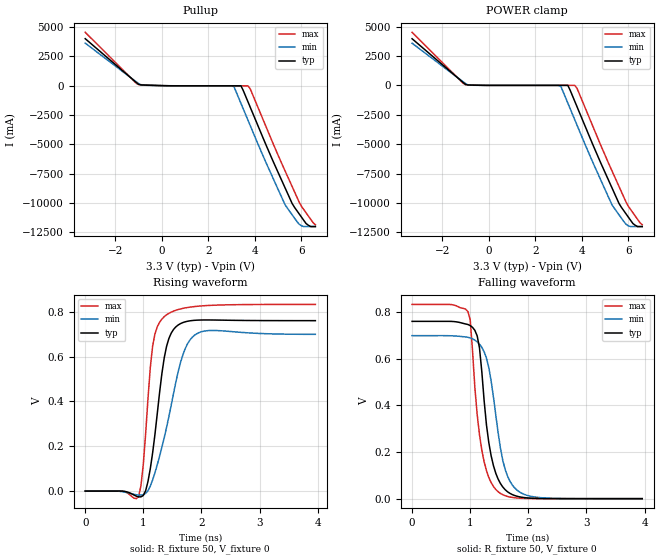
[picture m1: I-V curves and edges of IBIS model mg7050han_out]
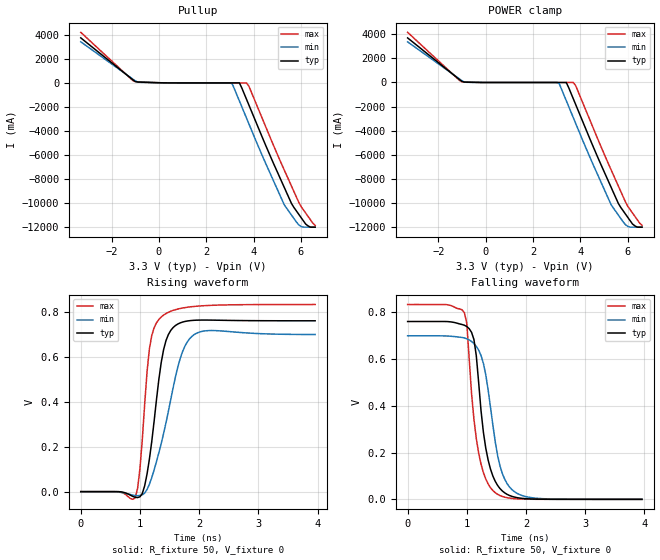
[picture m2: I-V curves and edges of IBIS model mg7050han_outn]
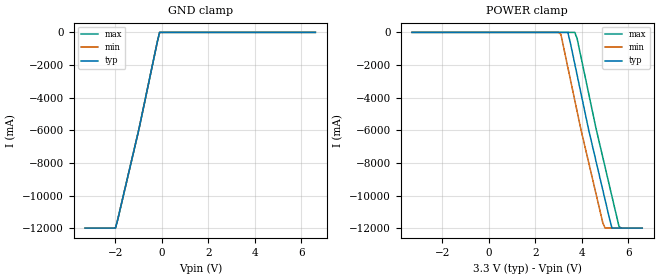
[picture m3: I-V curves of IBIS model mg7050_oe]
|   IBIS File mg7050han_4a_33v_100.ibs  ZSEL=H(ZO=100ohm)
[IBIS Ver]   3.2
[Comment Char]   |_char
[File name]   mg7050han_4a_33v_100.ibs
[File Rev]   1.0
[Date]   Jan 23, 2014
[Source]
|   Component MG7050HAN HCSL 4-OUTPUT 3.3V
[Component]   mg7050han-hcsl-4out-100ohm
[Manufacturer]   Seiko Epson Corporation
[Package]
| variable   typ   min   max
R_pkg   0.27   NA   NA
L_pkg   1.66n   NA   NA
C_pkg   0.53p   NA   NA
[Pin]   signal_name   model_name   R_pin   L_pin   C_pin
1   vcc1   POWER   NA   NA   NA
2   out1p   mg7050han_out   0.34   2.1nH   0.58pF
3   out1n   mg7050han_outn  0.25   1.5nH   0.50pF
4   out2p   mg7050han_out   0.22   1.3nH   0.44pF
5   out2n   mg7050han_outn  0.25   1.7nH   0.59pF
6   zsel   mg7050_zsel   NA   NA   NA
7   oe   mg7050_oe   NA   NA   NA
8   out3n   mg7050han_outn  0.25   1.7nH   0.62pF
9   out3p   mg7050han_out   0.22   1.3nH   0.49pF
10   out4n   mg7050han_outn  0.25   1.5nH   0.46pF
11   out4p   mg7050han_out   0.34   2.1nH   0.57pF
12   vcc2   POWER   NA   NA   NA
13   vcc   POWER   NA   NA   NA
14   gnd   GND   NA   NA   NA
[Diff Pin] inv_pin vdiff   tdelay_typ
2   3   0   0
4   5   0   0
9   8   0   0
11   10   0   0
| Models and submodels in the file (4): mg7050han_out (Open_source), mg7050han_outn (Open_source), mg7050_oe (Input), mg7050_zsel (Input)
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[Model]   mg7050han_out
Model_type Open_source
Enable Active-High
Polarity Non-Inverting
Vref=0
Vmeas=0.375
Rref=50
Cref=0
C_comp   4.79p   4.56p   5.00p
[Temperature Range] 25   85   -40
[Voltage Range]   3.3   2.97   3.63
[POWER Clamp Reference]3.3   2.97   3.63
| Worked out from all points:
|   slope of the pullup table from 0 to 0.495 V, typ, clamps not added: 36.3 ohm
|   POWER clamp passes 1 mA (typ) near -0.12 V on its own axis
|   falling waveform, R_fixture 50, V_fixture 0: 20-80 % time 215ps typ, 264ps min, 203ps max; typ from 0.761 V to 0 V
|   rising waveform, R_fixture 50, V_fixture 0: 20-80 % time 221ps typ, 363ps min, 161ps max; typ from 0 V to 0.761 V
[Pullup]
-3.3V     4.003A     3.625A     4.547A
-1V       105.9mA    168.5mA    94.6mA
3V        -15.26mA   -14.11mA   -16.67mA
3.1V      -15.26mA   -92.55mA   -16.7mA
3.4V      -15.27mA   -1.516A    -16.77mA
3.7V      -1.374A    -2.939A    -16.79mA
3.8V      -1.849A    -3.414A    -283.8mA
5.3V      -8.729A    -10.17A    -7.282A
5.6V      -10.05A    -11.01A    -8.598A
6V        -11.2A     -11.95A    -10.28A
6.3V      -11.91A    -12.01A    -11.12A
6.6V      -12.02A    -12.01A    -11.87A
[POWER Clamp]
-3.3V     3.964A     3.584A     4.512A
-1V       82.86mA    152.1mA    62.75mA
3V        -215.5pA   -247.8pA   -192.8pA
3.1V      -226.7pA   -83.17mA   -204pA
3.4V      -260.3pA   -1.507A    -237.6pA
3.7V      -1.364A    -2.93A     -271.3pA
3.8V      -1.839A    -3.405A    -272.9mA
5.3V      -8.719A    -10.16A    -7.271A
5.6V      -10.03A    -11A       -8.587A
6V        -11.19A    -11.94A    -10.27A
6.3V      -11.89A    -12A       -11.11A
6.6V      -12A       -12A       -11.85A
[Falling Waveform]
R_fixture=50
V_fixture=0
V_fixture_min=0
V_fixture_max=0
0s        760.7mV    699.5mV    833.4mV
960ps     747.2mV    692.4mV    802.9mV
1ns       742.6mV    689.8mV    767.4mV
1.12ns    698.5mV    672.8mV    361.2mV
1.2ns     544.1mV    648.9mV    208.1mV
1.32ns    240.8mV    562.5mV    91.12mV
1.48ns    84.18mV    283.9mV    29.88mV
1.64ns    30.11mV    98.17mV    9.663mV
1.92ns    4.964mV    19.44mV    1.33mV
3.96ns    0V         2.633uV    0V
[Rising Waveform]
R_fixture=50
V_fixture=0
V_fixture_min=0
V_fixture_max=0
0s        851.7nV    1.086uV    0V
920ps     -26.05mV   -17.89mV   -23.44mV
1ns       -19.53mV   -15.94mV   120.9mV
1.12ns    100.1mV    22.23mV    551.4mV
1.16ns    170.5mV    49.57mV    646.9mV
1.36ns    595.2mV    238.7mV    778.6mV
1.48ns    705.2mV    383.7mV    798.9mV
1.64ns    747.6mV    574.2mV    813.2mV
1.88ns    762.3mV    695.6mV    823.7mV
3.96ns    760.7mV    699.6mV    833.3mV
[Ramp]
R_load=50
dV/dt_r   4.564E-1/2.190E-10   4.197E-1/3.615E-10   5.000E-1/1.571E-10
dV/dt_f   4.564E-1/2.120E-10   4.197E-1/2.622E-10   5.000E-1/1.998E-10
|[End   mg7050han_out
[Model]   mg7050han_outn
Model_type Open_source
Enable Active-High
Polarity Inverting
Vref=0
Vmeas=0.375
Rref=50
Cref=0
C_comp   4.79p   4.56p   5.00p
[Temperature Range] 25   85   -40
[Voltage Range]   3.3   2.97   3.63
[POWER Clamp Reference]3.3   2.97   3.63
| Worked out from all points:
|   slope of the pullup table from 0 to 0.495 V, typ, clamps not added: 36.3 ohm
|   POWER clamp passes 1 mA (typ) near -0.12 V on its own axis
|   falling waveform, R_fixture 50, V_fixture 0: 20-80 % time 214ps typ, 266ps min, 204ps max; typ from 0.761 V to 0 V
|   rising waveform, R_fixture 50, V_fixture 0: 20-80 % time 219ps typ, 359ps min, 161ps max; typ from 0 V to 0.761 V
[Pullup]
-3.3V     3.733A     3.407A     4.193A
-1V       101.7mA    158.4mA    93.78mA
3V        -15.26mA   -14.11mA   -16.67mA
3.1V      -15.26mA   -92.55mA   -16.7mA
3.4V      -15.27mA   -1.516A    -16.77mA
3.7V      -1.374A    -2.939A    -16.79mA
3.8V      -1.849A    -3.414A    -283.8mA
5.3V      -8.729A    -10.17A    -7.282A
5.6V      -10.05A    -11.01A    -8.598A
6V        -11.2A     -11.95A    -10.28A
6.3V      -11.91A    -12.01A    -11.12A
6.6V      -12.02A    -12.01A    -11.87A
[POWER Clamp]
-3.3V     3.698A     3.37A      4.161A
-1V       79.16mA    143mA      62.06mA
3V        -215.5pA   -247.8pA   -192.9pA
3.1V      -226.7pA   -83.17mA   -204.1pA
3.4V      -260.3pA   -1.507A    -237.7pA
3.7V      -1.364A    -2.93A     -271.2pA
3.8V      -1.839A    -3.405A    -272.9mA
5.3V      -8.719A    -10.16A    -7.271A
5.6V      -10.03A    -11A       -8.587A
6V        -11.19A    -11.94A    -10.27A
6.3V      -11.9A     -12A       -11.11A
6.6V      -12A       -12A       -11.85A
[Falling Waveform]
R_fixture=50
V_fixture=0
V_fixture_min=0
V_fixture_max=0
0s        760.7mV    699.5mV    833.4mV
960ps     744.7mV    690.3mV    798.1mV
1ns       739mV      686.8mV    751.8mV
1.12ns    684mV      666.4mV    343.3mV
1.2ns     500.1mV    638.2mV    198.1mV
1.32ns    219.3mV    532.8mV    86.82mV
1.48ns    77.12mV    246.6mV    28.48mV
1.64ns    27.66mV    86.06mV    9.212mV
1.92ns    4.566mV    17.44mV    1.27mV
3.96ns    0V         2.43uV     0V
[Rising Waveform]
R_fixture=50
V_fixture=0
V_fixture_min=0
V_fixture_max=0
0s        -5.258uV   3.852uV    0V
920ps     -25.24mV   -17.29mV   -27.42mV
1ns       -23.01mV   -17.25mV   102.3mV
1.08ns    26.15mV    -6.425mV   388.9mV
1.16ns    145.1mV    33.14mV    636.4mV
1.24ns    314.9mV    97.2mV     730.1mV
1.4ns     632.9mV    259.3mV    786.3mV
1.68ns    751.4mV    592.8mV    815.6mV
1.92ns    763.1mV    700mV      824.8mV
3.96ns    760.8mV    699.7mV    833.3mV
[Ramp]
R_load=50
dV/dt_r   4.564E-1/2.174E-10   4.197E-1/3.584E-10   5.000E-1/1.562E-10
dV/dt_f   4.564E-1/2.126E-10   4.197E-1/2.634E-10   5.000E-1/2.000E-10
|[End   mg7050han_outn
[Model]   mg7050_oe
Model_type Input
Vinh=2.31
Vinl=0.99
C_comp   3p   3p   3p
[Temperature Range] 25   85   -40
[Voltage Range]   3.3   2.97   3.63
[POWER Clamp Reference]3.3   2.97   3.63
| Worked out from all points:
|   GND clamp passes 1 mA (typ) near -0.10 V on its own axis
[GND Clamp]
-3.3V     -12A       -12A       -12A
-2V       -12A       -12A       -12A
-1.9V     -11.47A    -11.47A    -11.47A
-1V       -6A        -6A        -6A
-200mV    -592.5mA   -592.5mA   -592.5mA
-100mV    -33.15uA   -29.16uA   -40.33uA
6.6V      32.19uA    34.53uA    32.12uA
[POWER Clamp]
-3.3V     32.19uA    31.39uA    35.69uA
3V        -29.25uA   -28.49uA   -32.44uA
3.1V      -30.22uA   -118.5mA   -33.52uA
3.4V      -33.15uA   -2.15A     -36.76uA
3.7V      -1.947A    -4.181A    -40uA
3.8V      -2.624A    -4.859A    -389.4mA
4.3V      -6A        -8.004A    -3.775A
4.9V      -9.645A    -11.65A    -7.64A
5V        -10.25A    -12A       -8.248A
5.3V      -12A       -12A       -10.07A
5.6V      -12A       -12A       -11.89A
6.6V      -12A       -12A       -12A
